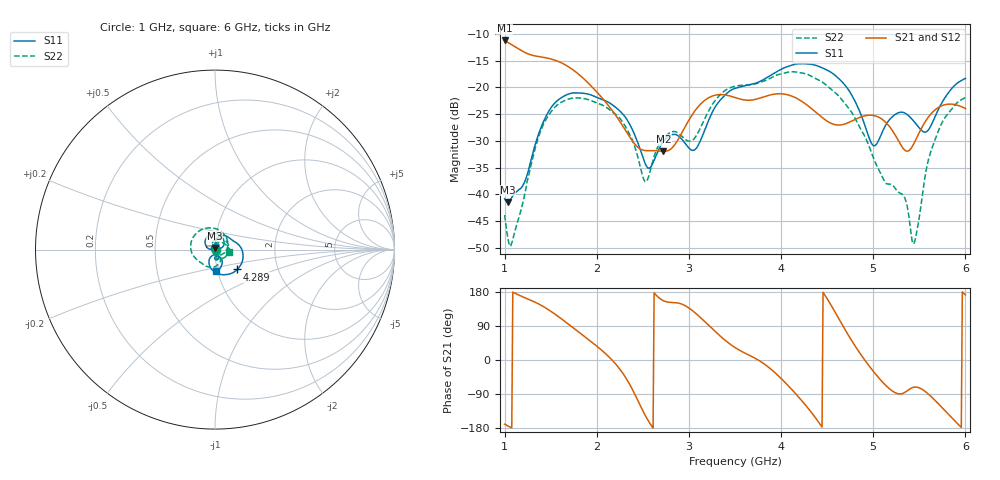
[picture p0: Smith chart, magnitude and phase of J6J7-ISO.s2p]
!Agilent Technologies,E8364B,MY43040528,A.07.50.67
!Agilent E8364B: A.07.50.67
!Date: Sunday, March 01, 2026 21:26:31
!Correction: S11(Full 2 Port(1,2))
!S21(Full 2 Port(1,2))
!S12(Full 2 Port(1,2))
!S22(Full 2 Port(1,2))
!S2P File: Measurements: S11, S21, S12, S22:
# Hz S  dB  R 50
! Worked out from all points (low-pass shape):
!   451 points, 1 GHz to 6 GHz, reference 50 ohm
!   highest |S21| = -11.21 dB at 1 GHz (marker M1); lowest = -32.0 dB at 2.722 GHz (marker M2)
!   |S21| within 3 dB of the highest: start of sweep to 1.364 GHz
!   lowest |S11| = -41.4 dB at 1.033 GHz (marker M3), VSWR 1.02, Z = 49.9 + j0.836 ohm
!   |S11| at or under -10 dB: start of sweep to end of sweep
!   |S22| runs from -49.7 to -17.1 dB; largest |S21 - S12| = 0.0011
!   S11 on the Smith chart (normalised r, x): 1 GHz: 1.00, +0.02; 4.289 GHz: 1.25, -0.28; 6 GHz: 0.98, -0.24
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1e9  -40.82 78.4  -11.21 -169.3  -11.25 -169.3  -43.87 2.1
1.033333e9  -41.44 98.6  -11.55 -173.7  -11.58 -173.7  -48.02 18.3
1.088889e9  -40.28 122.6  -12.13 179.2  -12.16 179.2  -48.47 61.9
1.222222e9  -37.46 156.2  -13.48 164.0  -13.51 164.0  -39.68 125.6
1.444444e9  -25.56 159.3  -14.44 137.5  -14.47 137.5  -26.14 98.7
1.844444e9  -21.08 87.2  -18.14 66.3  -18.17 66.3  -22.04 0.5
2.266667e9  -24.68 30.4  -26.79 -29.6  -26.81 -29.6  -26.12 -77.1
2.522222e9  -34.10 26.0  -31.80 -144.5  -31.84 -144.5  -37.59 -70.2
2.666667e9  -31.82 69.4  -31.87 165.8  -31.90 165.9  -30.93 -37.2
2.722222e9  -30.12 68.4  -31.95 156.5  -31.98 156.6  -29.54 -44.2
3.066667e9  -31.62 70.1  -24.34 124.6  -24.37 124.6  -29.37 -57.0
3.288889e9  -23.54 80.4  -21.43 74.3  -21.47 74.4  -22.34 -69.1
3.5e9  -20.18 50.5  -21.89 32.9  -21.92 32.9  -19.79 -108.0
4.288889e9  -15.61 -41.8  -23.39 -126.1  -23.43 -126.1  -17.58 118.0
4.344444e9  -15.72 -50.5  -24.16 -143.3  -24.20 -143.2  -18.06 105.0
4.711111e9  -19.95 -105.8  -26.72 73.2  -26.76 73.3  -23.41 5.2
5e9  -30.86 -94.5  -25.24 -29.6  -25.27 -29.6  -33.11 -115.4
5.166667e9  -26.23 -66.4  -27.11 -74.0  -27.15 -74.0  -38.09 127.6
5.333333e9  -24.72 -84.2  -31.58 -86.8  -31.61 -86.7  -40.33 22.6
5.444444e9  -26.39 -92.1  -30.39 -71.6  -30.42 -71.6  -49.08 -95.2
5.655556e9  -26.07 -57.4  -24.43 -103.0  -24.47 -102.9  -30.47 97.5
6e9  -18.32 -88.4  -23.94 171.9  -23.97 171.9  -21.90 -8.3
